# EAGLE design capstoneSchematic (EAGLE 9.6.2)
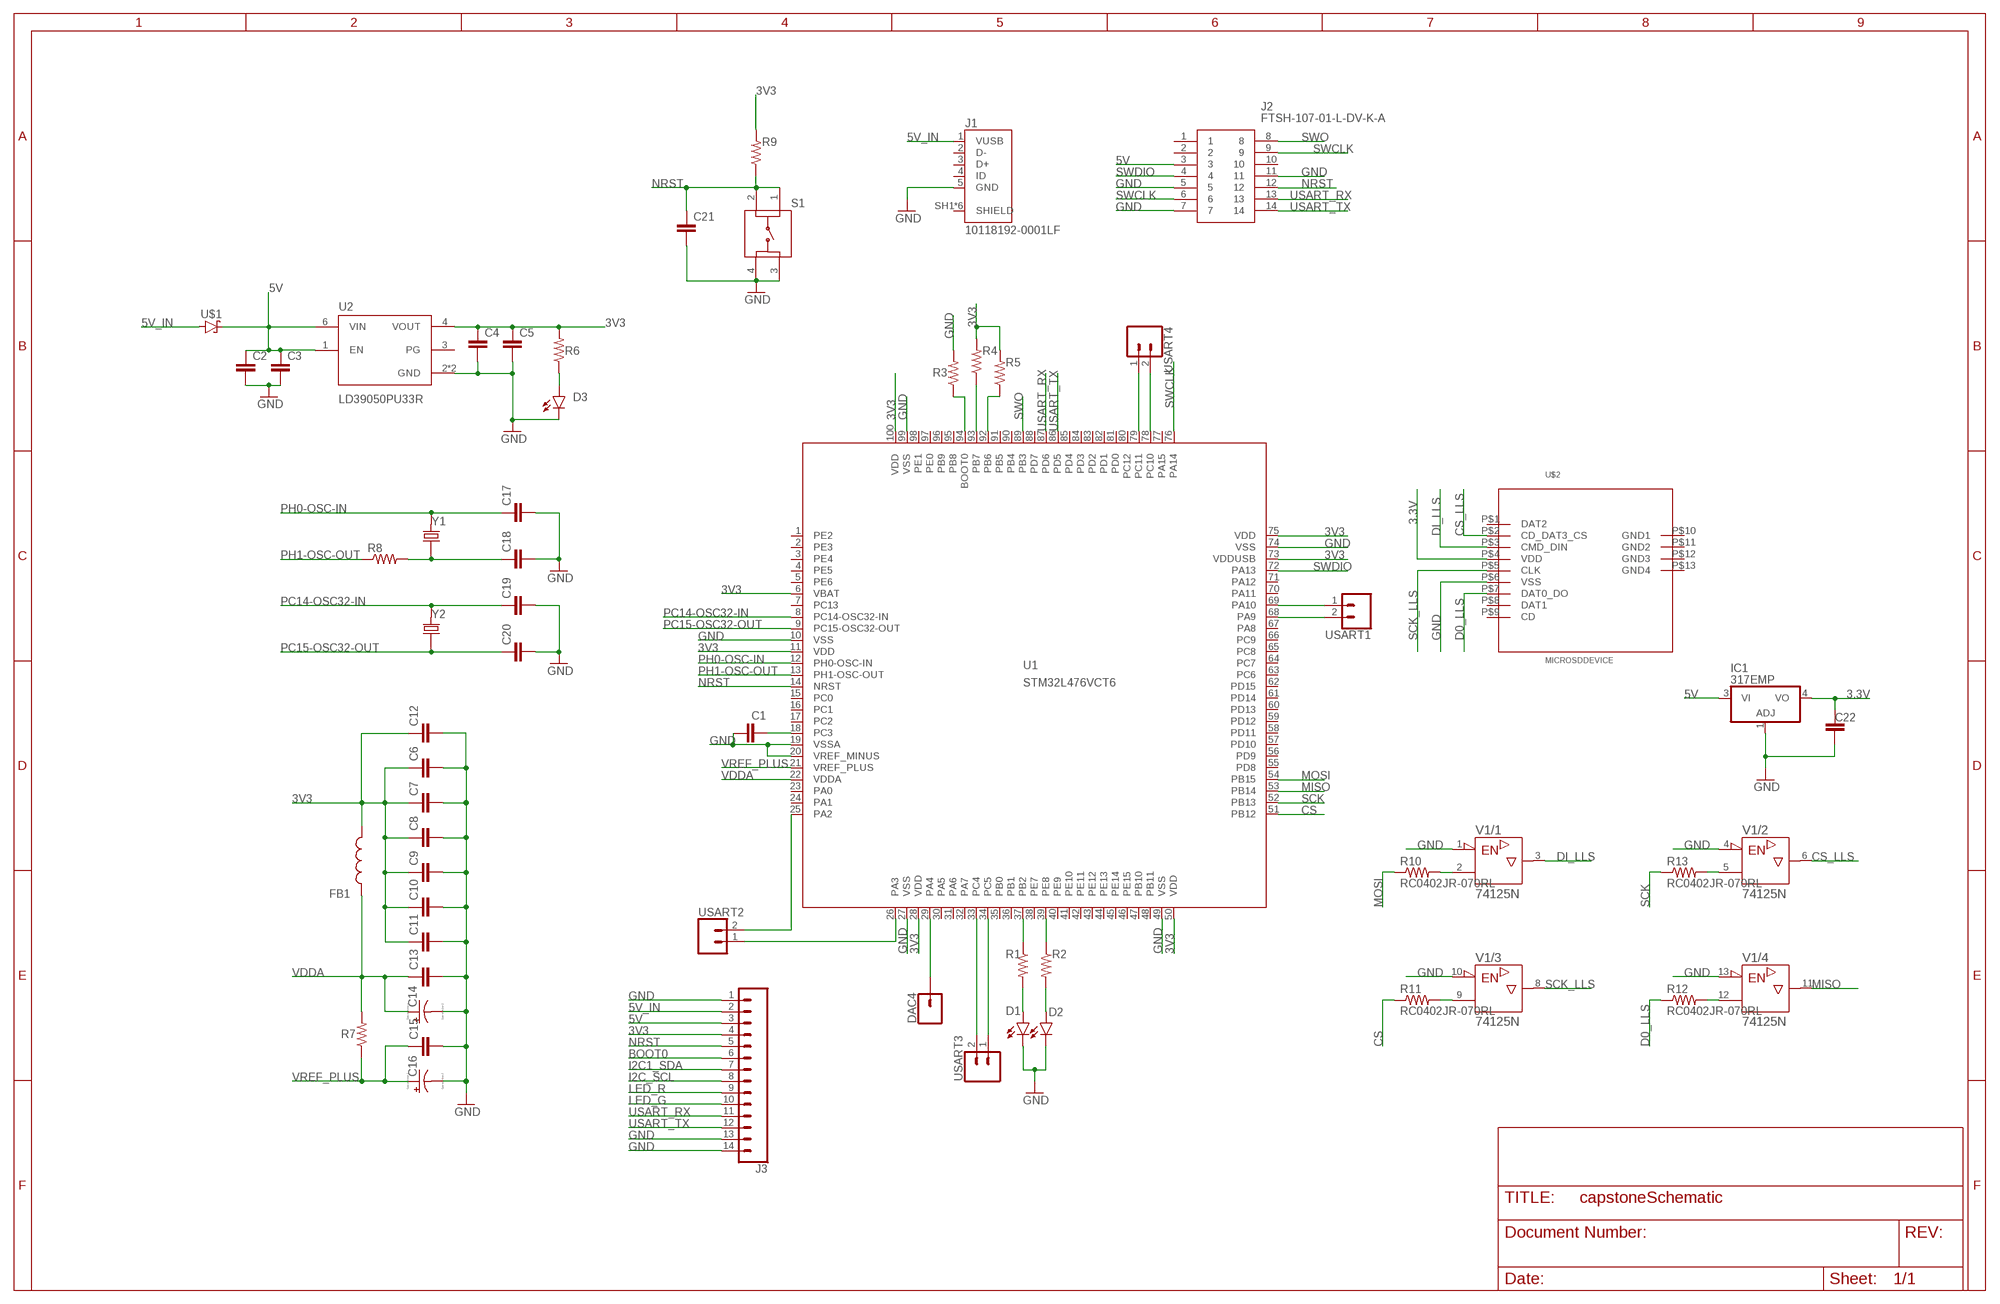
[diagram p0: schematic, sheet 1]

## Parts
C1  CC0603KRX5R7BB105  [CAPC1608X90]
C2  CC0603KRX5R7BB105  [CAPC1608X90]
C3  CC0402KRX7R7BB104  [CAPC1005X55N]
C4  CC0603KRX5R7BB105  [CAPC1608X90]
C5  CC0402KRX7R7BB104  [CAPC1005X55N]
C6  CC0402KRX7R7BB104  [CAPC1005X55N]
C7  CC0402KRX7R7BB104  [CAPC1005X55N]
C8  CC0402KRX7R7BB104  [CAPC1005X55N]
C9  CC0402KRX7R7BB104  [CAPC1005X55N]
C10  CC0402KRX7R7BB104  [CAPC1005X55N]
C11  CC0402KRX7R7BB104  [CAPC1005X55N]
C12  CC0603KRX5R7BB105  [CAPC1608X90]
C13  CC0402KRX7R7BB104  [CAPC1005X55N]
C14  TAJA105K016RNJ  [CAPPM3216X180N]
C15  CC0402KRX7R7BB104  [CAPC1005X55N]
C16  TAJA105K016RNJ  [CAPPM3216X180N]
C17  CC0402JRNPO9BN200  [CAPC1005X55N]
C18  CC0402JRNPO9BN200  [CAPC1005X55N]
C19  CC0402CRNPO9BN4R7  [CAPC1005X55N]
C20  CC0402CRNPO9BN4R7  [CAPC1005X55N]
C21  CC0402KRX7R7BB104  [CAPC1005X55N]
C22  C  (no package)
D1  SML-P12MTT86  [LED_SML-P11UTT86R]
D2  SML-P12MTT86  [LED_SML-P11UTT86R]
D3  SML-P12MTT86  [LED_SML-P11UTT86R]
DAC4  CONN_01  [1X01]
FB1  BK1608HS601-T  [BEADC1608X95N]
IC1  317EMP  [SOT223]
J1  10118192-0001LF  [AMPHENOL_10118192-0001LF]
J2  FTSH-107-01-L-DV-K-A  [FTSH10701LDVKA]
J3  CONN_14  [1X14]
R1  RC0402FR-071KL  [RESC1005X40N]
R2  RC0402FR-071KL  [RESC1005X40N]
R3  RC0402FR-071KL  [RESC1005X40N]
R4  RC0402FR-071KL  [RESC1005X40N]
R5  RC0402FR-071KL  [RESC1005X40N]
R6  RC0402FR-071KL  [RESC1005X40N]
R7  RC0402FR-071KL  [RESC1005X40N]
R8  RC0402FR-072KL  [RESC1005X40N]
R9  RC0402FR-0710KL  [RESC1005X40N]
R10  RC0402JR-070RL  [RESC1005X40]
R11  RC0402JR-070RL  [RESC1005X40]
R12  RC0402JR-070RL  [RESC1005X40]
R13  RC0402JR-070RL  [RESC1005X40]
S1  LL3301FF065QJ  [LL3301FF065QJ]
U1  STM32L476VCT6  [LQFP100_14X14]
U2  LD39050PU33R  [SON95P300X300X100-7N]
U$1  STPS1L30A  [DIOM5226X223N]
U$2  MICROSDDEVICE  [MICROSD]
USART1  CONN_02  [1X02]
USART2  CONN_02  [1X02]
USART3  CONN_02  [1X02]
USART4  CONN_02  [1X02]
V1  74125N  [DIL14]
Y1  ABLS-8.000MHZ-B2-T  [XTAL_ABLS-8.000MHZ-B2-T]
Y2  ECS-.327-12.5-12QS-TR  [XTAL_ECS-.327-12.5-12QS-TR]

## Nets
3.3V: C22.1 IC1.4(VO) U$2.P$4(VDD)
3V3: C4.1 C5.1 C6.1 C7.1 C8.1 C9.1 C10.1 C11.1 C12.1 FB1.2 J3.4 R4.2 R5.2 R6.2 R9.2 U1.6(VBAT) U1.11(VDD) U1.28(VDD) U1.50(VDD) U1.73(VDDUSB) U1.75(VDD) U1.100(VDD) U2.4(VOUT)
5V: C2.1 C3.1 IC1.3(VI) J2.3 J3.3 U2.1(EN) U2.6(VIN) U$1.1(C)
5V_IN: J1.1(VUSB) J3.2 U$1.2(A)
BOOT0: J3.6
CS: R11.1 U1.51(PB12)
CS_LLS: U$2.P$2(CD_DAT3_CS) V1.6(/2:Y)
D0_LLS: R12.1 U$2.P$7(DAT0_DO)
DI_LLS: U$2.P$3(CMD_DIN) V1.3(/1:Y)
GND: C1.1 C2.2 C3.2 C4.2 C5.2 C6.2 C7.2 C8.2 C9.2 C10.2 C11.2 C12.2 C13.2 C14.C(-) C15.2 C16.C(-) C17.2 C18.2 C19.2 C20.2 C21.2 C22.2 D1.C D2.C D3.C IC1.1(ADJ) J1.5(GND) J2.5 J2.7 J2.11 J3.1 J3.13 J3.14 R3.2 S1.3 S1.4 U1.10(VSS) U1.19(VSSA) U1.20(VREF_MINUS) U1.27(VSS) U1.49(VSS) U1.74(VSS) U1.99(VSS) U2.2(GND) U2.7(GND) U$2.P$6(VSS) V1.1(/1:!G) V1.4(/2:!G) V1.10(/3:!G) V1.13(/4:!G)
I2C1_SDA: J3.7
I2C_SCL: J3.8
LED_G: J3.10
LED_R: J3.9
MISO: U1.53(PB14) V1.11(/4:Y)
MOSI: R10.1 U1.54(PB15)
N$1: R2.1 U1.39(PE8)
N$2: R1.1 U1.37(PB2)
N$3: D1.A R1.2
N$4: D2.A R2.2
N$5: R3.1 U1.94(BOOT0)
N$6: R4.1 U1.93(PB7)
N$7: R5.1 U1.92(PB6)
N$8: D3.A R6.1
N$9: U1.33(PC4) USART3.2
N$10: C1.2 U1.18(PC3)
N$11: U1.34(PC5) USART3.1
N$12: C18.1 R8.2 Y1.1
N$13: R10.2 V1.2(/1:A)
N$14: U1.78(PC10) USART4.2
N$15: R11.2 V1.9(/3:A)
N$16: U1.79(PC11) USART4.1
N$17: R13.2 V1.5(/2:A)
N$18: DAC4.1 U1.29(PA4)
N$19: U1.69(PA10) USART1.1
N$20: U1.68(PA9) USART1.2
N$21: R12.2 V1.12(/4:A)
N$22: U1.25(PA2) USART2.2
N$23: U1.26(PA3) USART2.1
NRST: C21.1 J2.12 J3.5 R9.1 S1.1 S1.2 U1.14(NRST)
PC14-OSC32-IN: C19.1 U1.8(PC14-OSC32-IN) Y2.2
PC15-OSC32-OUT: C20.1 U1.9(PC15-OSC32-OUT) Y2.1
PH0-OSC-IN: C17.1 U1.12(PH0-OSC-IN) Y1.2
PH1-OSC-OUT: R8.1 U1.13(PH1-OSC-OUT)
SCK: R13.1 U1.52(PB13)
SCK_LLS: U$2.P$5(CLK) V1.8(/3:Y)
SWCLK: J2.6 J2.9 U1.76(PA14)
SWDIO: J2.4 U1.72(PA13)
SWO: J2.8 U1.89(PB3)
USART_RX: J2.13 J3.11 U1.87(PD6)
USART_TX: J2.14 J3.12 U1.86(PD5)
VDDA: C13.1 C14.A(+) FB1.1 R7.2 U1.22(VDDA)
VREF_PLUS: C15.1 C16.A(+) R7.1 U1.21(VREF_PLUS)
Unconnected: J1.2(D-) J1.3(D+) J1.4(ID) J1.SH1(SHIELD) J1.SH2(SHIELD) J1.SH3(SHIELD) J1.SH4(SHIELD) J1.SH5(SHIELD) J1.SH6(SHIELD) J2.1 J2.2 J2.10 U1.1(PE2) U1.2(PE3) U1.3(PE4) U1.4(PE5) U1.5(PE6) U1.7(PC13) U1.15(PC0) U1.16(PC1) U1.17(PC2) U1.23(PA0) U1.24(PA1) U1.30(PA5) U1.31(PA6) U1.32(PA7) U1.35(PB0) U1.36(PB1) U1.38(PE7) U1.40(PE9) U1.41(PE10) U1.42(PE11) U1.43(PE12) U1.44(PE13) U1.45(PE14) U1.46(PE15) U1.47(PB10) U1.48(PB11) U1.55(PD8) U1.56(PD9) U1.57(PD10) U1.58(PD11) U1.59(PD12) U1.60(PD13) U1.61(PD14) U1.62(PD15) U1.63(PC6) U1.64(PC7) U1.65(PC8) U1.66(PC9) U1.67(PA8) U1.70(PA11) U1.71(PA12) U1.77(PA15) U1.80(PC12) U1.81(PD0) U1.82(PD1) U1.83(PD2) U1.84(PD3) U1.85(PD4) U1.88(PD7) U1.90(PB4) U1.91(PB5) U1.95(PB8) U1.96(PB9) U1.97(PE0) U1.98(PE1) U2.3(PG) U$2.P$1(DAT2) U$2.P$8(DAT1) U$2.P$9(CD) U$2.P$10(GND1) U$2.P$11(GND2) U$2.P$12(GND3) U$2.P$13(GND4)

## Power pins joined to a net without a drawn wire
+UB: V1.14(/+UB:+UB)
-UB: V1.7(/-UB:-UB)

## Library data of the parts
C1 C2 C4 C12 = ce-capstone:CC0603KRX5R7BB105: CAPACITOR CERAMIC, 1µF, 10V, X5R, 0603; Dielectric Characteristic:X5R; Capacitance:1µF; Capacitance Tolerance:± 10%; Voltage Rating:16V; Temperature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; DESCRIPTION: 1µF ±10% 16V Ceramic Capacitor X5R 0603 _1608 Metric_; DIGI-KEY_PART_NUMBER: 311-1444-1-ND; DIGI-KEY_PURCHASE_URL: https://www.digikey.com/product-detail/en/yageo/CC0603KRX5R7BB105/311-1444-1-ND/2833750?utm_source=snapeda&utm_medium=aggregator&utm_campaign=symbol; MF: Yageo; MP: CC0603KRX5R7BB105; PACKAGE: 0603 Yageo
C3 C5-C11 C13 C15 C21 = ce-capstone:CC0402KRX7R7BB104: .1UF 16V 10% 0402; DESCRIPTION: 0.1µF ±10% 16V Ceramic Capacitor X7R 0402 _1005 Metric_; DIGI-KEY_PART_NUMBER: 311-1338-1-ND; DIGI-KEY_PURCHASE_URL: https://www.digikey.com/product-detail/en/yageo/CC0402KRX7R7BB104/311-1338-1-ND/2103122?utm_source=snapeda&utm_medium=aggregator&utm_campaign=symbol; MF: Yageo; MP: CC0402KRX7R7BB104; PACKAGE: 0402 Yageo
C14 C16 = ce-capstone:TAJA105K016RNJ: Capacitor tantalum TAJ 1206 1uF 16V AVX 1uF SMD Solid MnO2 Tantalum Electrolytic Capacitor, 16 V dc +/-10%, TAJ Series; ALLIED_NUMBER: 70474975; ALLIED_PRICE-STOCK: https://www.alliedelec.com/avx-taja105k016r/70474975/; DESCRIPTION: Capacitor tantalum TAJ 1206 1uF 16V AVX 1uF SMD Solid MnO2 Tantalum Electrolytic Capacitor, 16 V dc +/-10%, TAJ Series; HEIGHT: 1.8mm; MANUFACTURER_NAME: AVX; MANUFACTURER_PART_NUMBER: TAJA105K016RNJ; MOUSER_PART_NUMBER: 581-TAJA105K016RNJ; MOUSER_PRICE-STOCK: https://www.mouser.com/Search/Refine.aspx?Keyword=581-TAJA105K016R; RS_PART_NUMBER: 6992804P; RS_PRICE-STOCK: http://uk.rs-online.com/web/p/products/6992804P
C17 C18 = ce-capstone:CC0402JRNPO9BN200: CAPACITOR CERAMIC 20PF 50V, C0G, 0402; Dielectric Characteristic:C0G / NP0; Capacitance:20pF; Capacitance Tolerance:± 5%; Voltage Rating:50V; Capacitor Case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; DESCRIPTION: 20pF ±5% 50V Ceramic Capacitor C0G, NP0 0402 _1005 Metric_; DIGI-KEY_PART_NUMBER: 311-1417-1-ND; DIGI-KEY_PURCHASE_URL: https://www.digikey.com/product-detail/en/yageo/CC0402JRNPO9BN200/311-1417-1-ND/2833723?utm_source=snapeda&utm_medium=aggregator&utm_campaign=symbol; MF: Yageo; MP: CC0402JRNPO9BN200; PACKAGE: 0402 Yageo
C19 C20 = ce-capstone:CC0402CRNPO9BN4R7: 0402 4.7 pF 50 V ±0.25 pF Tolerance NP0 SMT Multilayer Ceramic Capacitor; DESCRIPTION: 4.7pF ±0.25pF 50V Ceramic Capacitor C0G, NP0 0402 _1005 Metric_; DIGI-KEY_PART_NUMBER: 311-1367-1-ND; DIGI-KEY_PURCHASE_URL: https://www.digikey.com/product-detail/en/yageo/CC0402CRNPO9BN4R7/311-1367-1-ND/2103151?utm_source=snapeda&utm_medium=aggregator&utm_campaign=symbol; MF: Yageo; MP: CC0402CRNPO9BN4R7; PACKAGE: 0402 Yageo
C22 = ngspice-simulation:C: CAPACITOR
D1-D3 = ce-capstone:SML-P12MTT86: SML-P1 Series Red 0402 Clear 60 mcd 2 V Surface Mount PICOLED LED; AVAILABILITY: Unavailable; DESCRIPTION: Green 572nm LED Indication - Discrete 2V 0402 _1006 Metric_; MF: Rohm; MP: SML-P12MTT86; PACKAGE: 0402 Rohm; PRICE: None
DAC4 = SparkFun-Connectors:CONN_01: Single connection point. Often used as Generic Header-pin footprint for 0.1 inch spaced/style header connections
FB1 = ce-capstone:BK1608HS601-T: Ferrite Chip Bead(Lead Free); DESCRIPTION: Ferrite Chip Bead(Lead Free); HEIGHT: 0.95mm; MANUFACTURER_NAME: Taiyo Yuden; MANUFACTURER_PART_NUMBER: BK1608HS601-T
IC1 = linear:*317: Positive VOLTAGE REGULATOR
J1 = ce-capstone:10118192-0001LF: Single Port 5 Contact Horizontal Right Angle Shielded Micro B USB 2.0 Connector; AVAILABILITY: Unavailable; DESCRIPTION: USB - micro B USB 2.0 Receptacle Connector 5 Position Surface Mount, Right Angle; MF: Amphenol ICC; MP: 10118192-0001LF; PACKAGE: None; PRICE: None
J2 = ce-capstone:FTSH-107-01-L-DV-K-A: Headers & Wire Housings .050" Micro Terminal Strip Source: Datasheet; DESCRIPTION: Headers & Wire Housings .050" Micro Terminal Strip; HEIGHT: 5.97mm; MANUFACTURER_NAME: SAMTEC; MANUFACTURER_PART_NUMBER: FTSH-107-01-L-DV-K-A; MOUSER_PART_NUMBER: 200-FTSH10701LDVKA; MOUSER_PRICE-STOCK: https://www.mouser.com/Search/Refine.aspx?Keyword=200-FTSH10701LDVKA
J3 = SparkFun-Connectors:CONN_14: Multi connection point. Often used as Generic Header-pin footprint for 0.1 inch spaced/style header connections On any of the 0.1 inch spaced packages, you can populate with these: Break Away Headers - Straight (PRT-00116) Break Away Male Headers - Right Angle (PRT-00553) Female Headers (PRT-00115)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
R1-R7 = ce-capstone:RC0402FR-071KL: RES SMD 1k OHM 1% 1/16W 0402; DESCRIPTION: 510 Ohms ±1% 0.063W, 1/16W Chip Resistor 0402 _1005 Metric_ Moisture Resistant Thick Film; DIGI-KEY_PART_NUMBER: 311-510LRCT-ND; DIGI-KEY_PURCHASE_URL: https://www.digikey.com/product-detail/en/yageo/RC0402FR-07510RL/311-510LRCT-ND/729579?utm_source=snapeda&utm_medium=aggregator&utm_campaign=symbol; MF: Yageo; MP: RC0402FR-07510RL; PACKAGE: 1005 Panasonic Electronic Components
R8 = ce-capstone:RC0402FR-072KL: RES SMD 2k OHM 1% 1/16W 0402; DESCRIPTION: 510 Ohms ±1% 0.063W, 1/16W Chip Resistor 0402 _1005 Metric_ Moisture Resistant Thick Film; DIGI-KEY_PART_NUMBER: 311-510LRCT-ND; DIGI-KEY_PURCHASE_URL: https://www.digikey.com/product-detail/en/yageo/RC0402FR-07510RL/311-510LRCT-ND/729579?utm_source=snapeda&utm_medium=aggregator&utm_campaign=symbol; MF: Yageo; MP: RC0402FR-07510RL; PACKAGE: 1005 Panasonic Electronic Components
R9 = ce-capstone:RC0402FR-0710KL: RES SMD 10k OHM 1% 1/16W 0402; DESCRIPTION: 510 Ohms ±1% 0.063W, 1/16W Chip Resistor 0402 _1005 Metric_ Moisture Resistant Thick Film; DIGI-KEY_PART_NUMBER: 311-510LRCT-ND; DIGI-KEY_PURCHASE_URL: https://www.digikey.com/product-detail/en/yageo/RC0402FR-07510RL/311-510LRCT-ND/729579?utm_source=snapeda&utm_medium=aggregator&utm_campaign=symbol; MF: Yageo; MP: RC0402FR-07510RL; PACKAGE: 1005 Panasonic Electronic Components
R10-R13 = ce-capstone:RC0402JR-070RL: RC Series 0402 62.5 mW 0 Ohms 5% ±200 ppm/°C SMT Thick Film Chip Resistor; AVAILABILITY: Unavailable; DESCRIPTION: 0 Ohms Jumper 0.063W, 1/16W Chip Resistor 0402 _1005 Metric_ Moisture Resistant Thick Film; MF: Yageo; MP: RC0402JR-070RL; PACKAGE: 0402 Yageo; PRICE: None
S1 = ce-capstone:LL3301FF065QJ: Pushbutton Switches 50mA 12VDC F065 7.0mm J-Lead Source: Datasheet; DESCRIPTION: Pushbutton Switches 50mA 12VDC F065 7.0mm J-Lead; HEIGHT: 7.3mm; MANUFACTURER_NAME: E-Switch; MANUFACTURER_PART_NUMBER: LL3301FF065QJ; MOUSER_PART_NUMBER: 612-LL3301FF065QJ; MOUSER_PRICE-STOCK: https://www.mouser.com/Search/Refine.aspx?Keyword=612-LL3301FF065QJ
U1 = ce-capstone:STM32L476V*: STM32L476VX LQFP100 Datasheet STM32L476XX; FARNELL: 2518171; FLASH: 256kB; SRAM: 128kB
U2 = ce-capstone:LD39050PU33R: LD39050 Series 500 mA 3.3 V Fixed Low Noise LDO Voltage Regulator - DFN-6; AVAILABILITY: Unavailable; DESCRIPTION: Linear Voltage Regulator IC 1 Output 500mA 6-DFN _3x3_; MF: STMicroelectronics; MP: LD39050PU33R; PACKAGE: DFN-6 STMicroelectronics; PRICE: None
U$1 = ce-capstone:STPS1L30A
U$2 = MicroSDFootprint:MICROSDDEVICE
USART1-USART4 = SparkFun-Connectors:CONN_02: Multi connection point. Often used as Generic Header-pin footprint for 0.1 inch spaced/style header connections
V1 = 74ttl-din:74*125: Quad bus BUFFER, 3-state
Y1 = ce-capstone:ABLS-8.000MHZ-B2-T: Crystal 8MHz Â±20ppm (Tol) Â±50ppm (Stability) 18pF FUND 80Ohm 2-Pin HC-49/US SMD T/R; AVAILABILITY: Unavailable; DESCRIPTION: 8MHz ±20ppm Crystal 18pF 80 Ohms HC-49/US; MF: Abracon LLC; MP: ABLS-8.000MHZ-B2; PACKAGE: HC-49/US Abracon LLC; PRICE: None
Y2 = ce-capstone:ECS-.327-12.5-12QS-TR: SMD CRYSTAL 32.768 KHz; AVAILABILITY: Unavailable; DESCRIPTION: 32.768kHz ±20ppm Crystal 12.5pF 90 kOhms 2-SMD, No Lead; MF: ECS Inc.; MP: ECS-.327-12.5-12QS-TR; PACKAGE: SMD-2 ECS International; PRICE: None

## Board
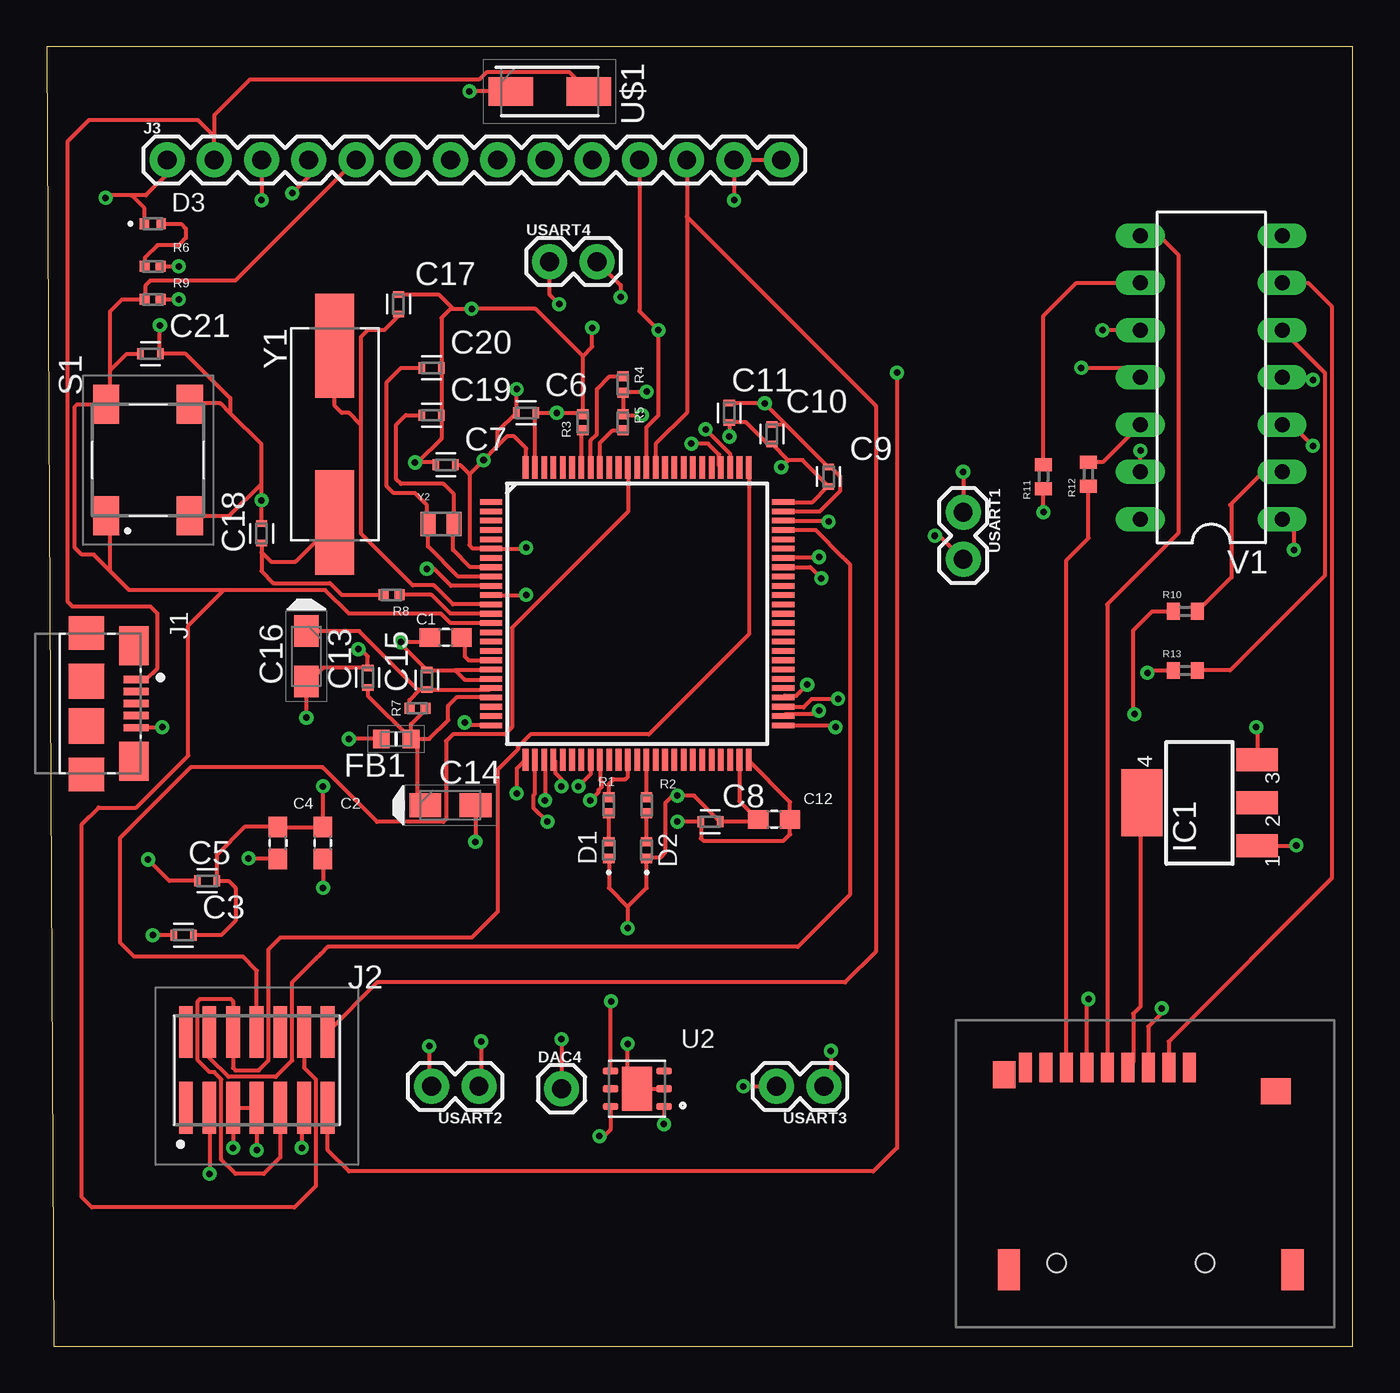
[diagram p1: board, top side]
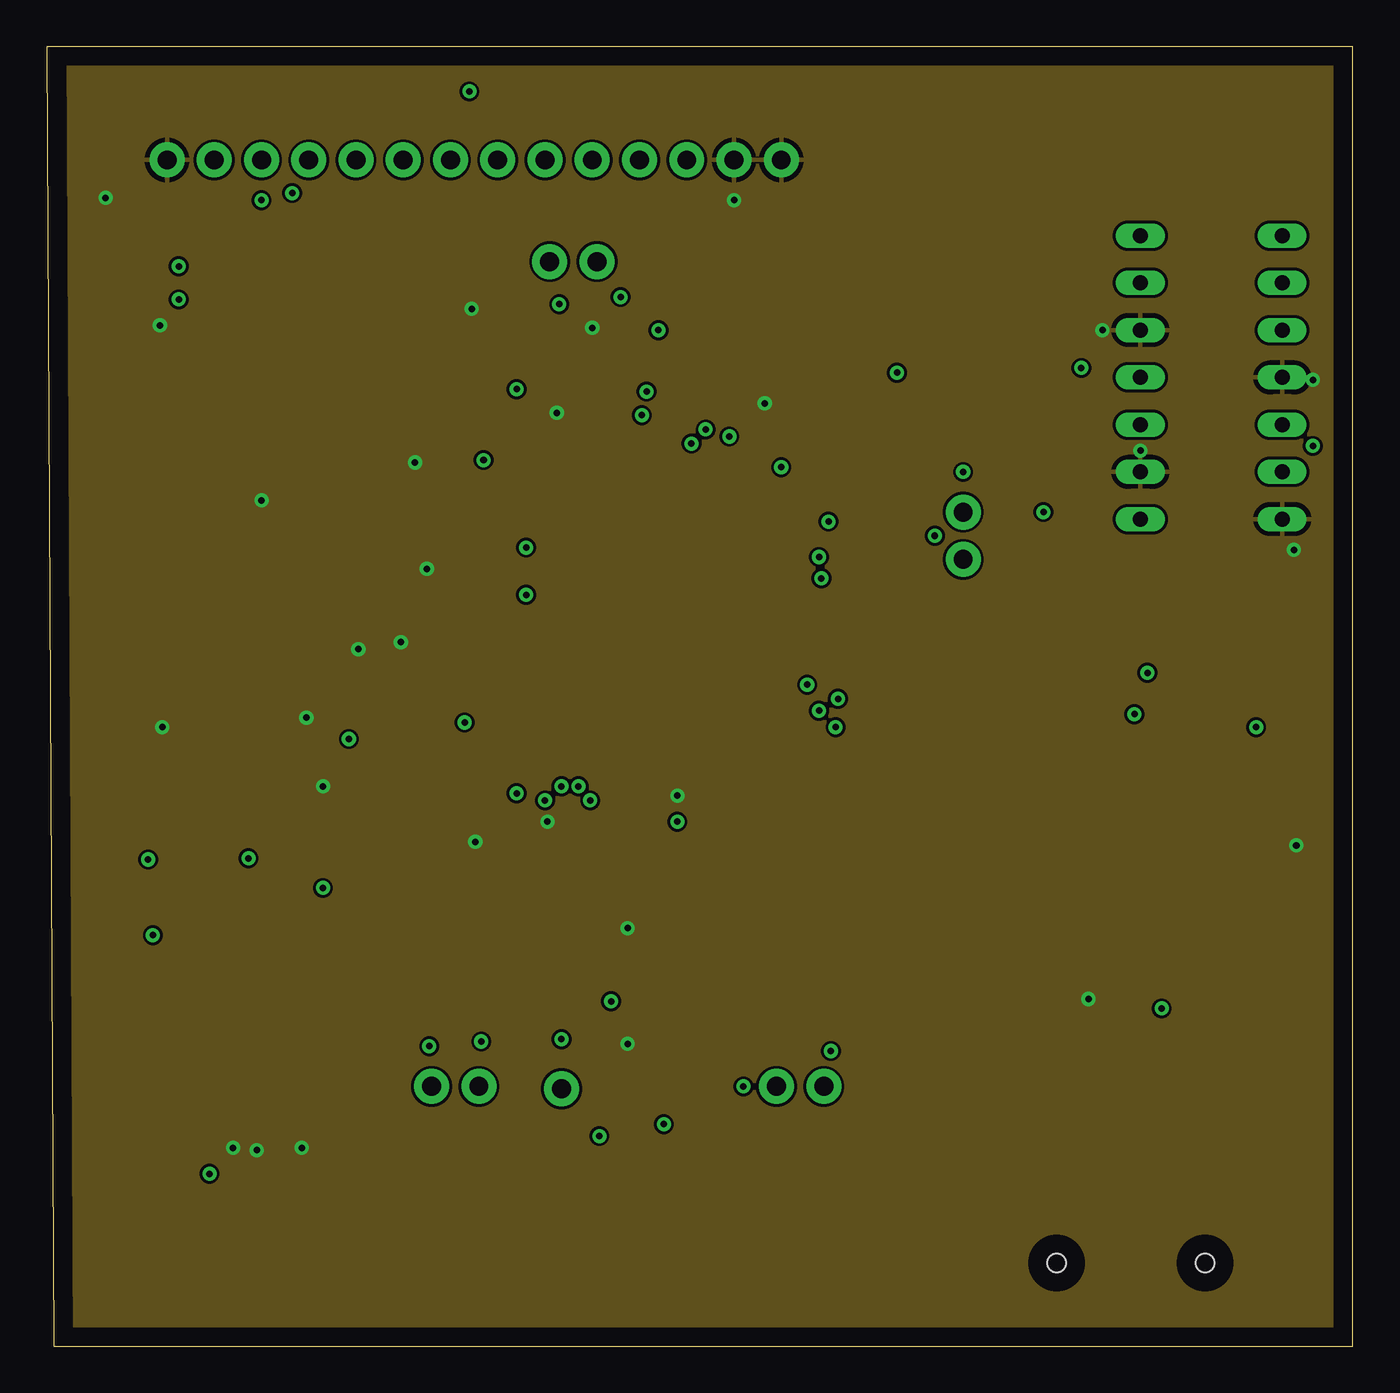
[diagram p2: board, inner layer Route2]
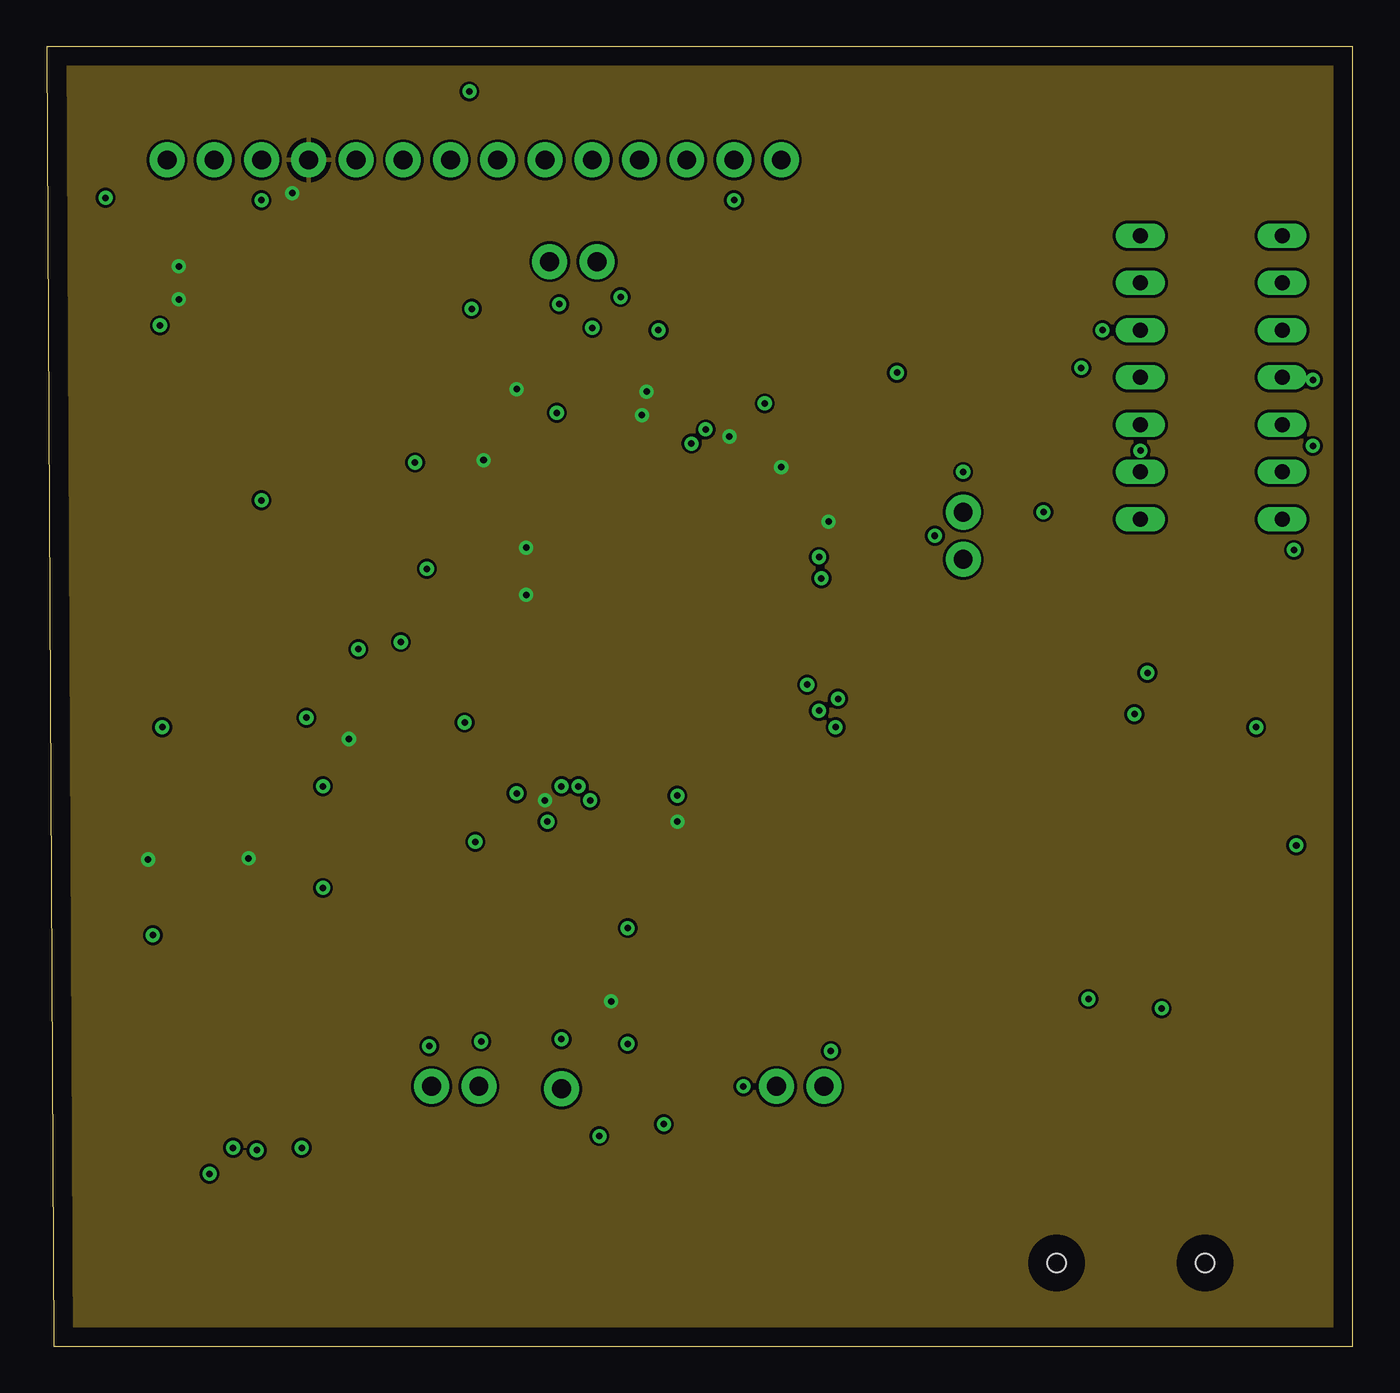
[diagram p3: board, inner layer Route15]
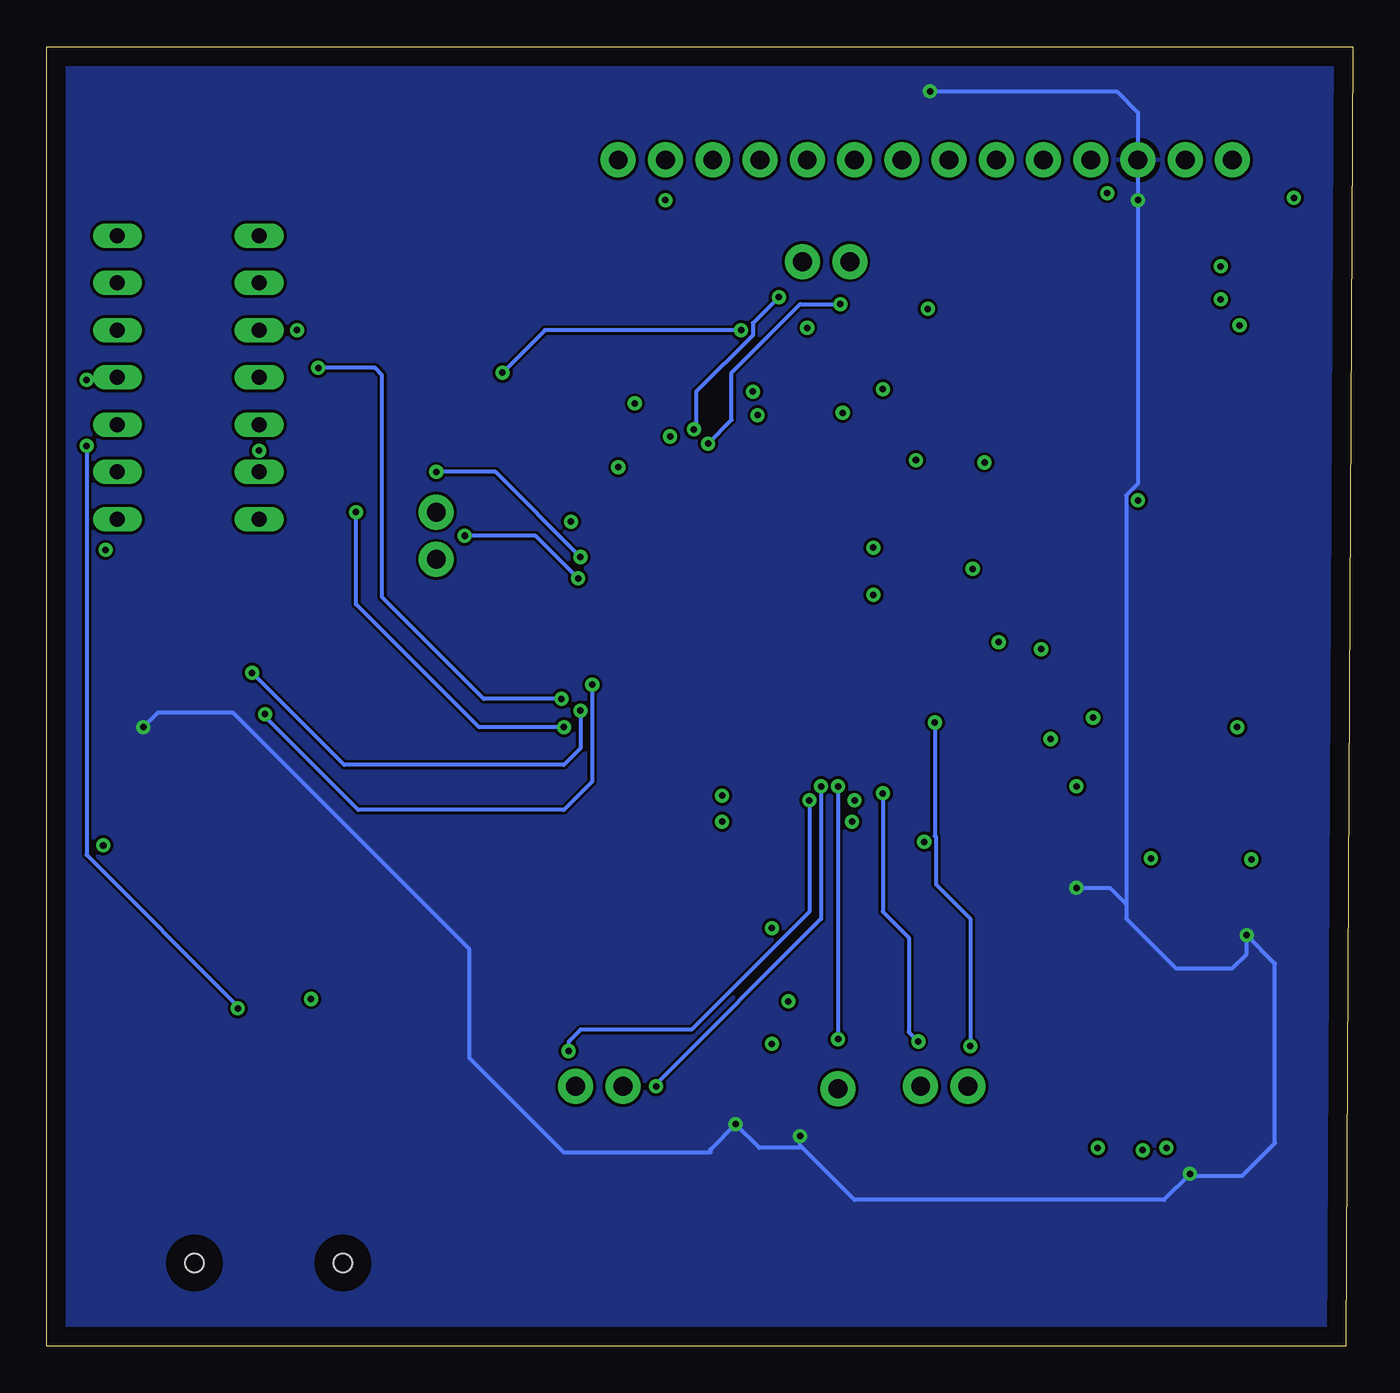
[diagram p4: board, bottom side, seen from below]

Size 70.23 x 69.85 mm. Coordinates in mm from the lower left corner, seen from the top.
Outline: 0.38,0 70.23,0 70.23,69.85 0,69.85 0.38,0
Copper layers (1+2*15+16): Top 0.035mm / dielectric 1.5mm / Route2 0.035mm / dielectric 0.15mm / Route15 0.035mm / dielectric 0.2mm / Bottom 0.035mm
Design rules "default *": minimum track width 8mil, minimum drill 0.35mm, track to track 6mil, track to pad 6mil, pad to pad 6mil, via to via 6mil, smd to smd 6mil, copper to edge 40mil, drill to drill 6mil, minimum pad ring 10mil, minimum via ring 8mil, stop-mask expansion 4mil, vias tented up to drill 0mil, thermal gap 10mil

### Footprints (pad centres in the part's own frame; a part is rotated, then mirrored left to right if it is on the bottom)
CAPC1608X90 = smd 1.1 x 1: 1 -0.85,0; 2 0.85,0
CAPC1005X55N = smd 0.35 x 0.6: 1 -0.525,0; 2 0.525,0
CAPPM3216X180N = smd 1.7 x 1.3: A -1.35,0; C 1.35,0
LED_SML-P11UTT86R = smd 0.5 x 0.6: A 0.45,0; C -0.45,0
1X01 = drill 1.016 pad 1.88: 1 0,0
BEADC1608X95N = smd 0.9 x 1: 1 -0.8,0; 2 0.8,0
SOT223 = smd 1.219 x 2.235: 1 -2.311,-3.099; 2 0,-3.099; 3 2.311,-3.099 | smd 3.6 x 2.2: 4 0,3.099
AMPHENOL_10118192-0001LF = smd 0.4 x 1.35: 1 -1.3,0; 2 -0.65,0; 3 0,0; 4 0.65,0; 5 1.3,0 | smd 2.1 x 1.6: SH1 -3.1,-0.125; SH2 3.1,-0.125 | smd 1.8 x 1.9: SH3 -3.8,-2.675; SH6 3.8,-2.675 | smd 1.9 x 1.9: SH4 -1.2,-2.675; SH5 1.2,-2.675
FTSH10701LDVKA = smd 0.74 x 2.79: 1 -3.81,-2.035; 2 -3.81,2.035; 3 -2.54,-2.035; 4 -2.54,2.035; 5 -1.27,-2.035; 6 -1.27,2.035; 7 0,-2.035; 8 0,2.035; 9 1.27,-2.035; 10 1.27,2.035; 11 2.54,-2.035; 12 2.54,2.035; 13 3.81,-2.035; 14 3.81,2.035
1X14 = drill 1.016 pad 1.88: 1 0,0; 2 2.54,0; 3 5.08,0; 4 7.62,0; 5 10.16,0; 6 12.7,0; 7 15.24,0; 8 17.78,0; 9 20.32,0; 10 22.86,0; 11 25.4,0; 12 27.94,0; 13 30.48,0; 14 33.02,0
RESC1005X40N = smd 0.54 x 0.6: 1 -0.432,0; 2 0.432,0
RESC1005X40 = smd 0.7 x 0.9: 1 -0.65,0; 2 0.65,0
LL3301FF065QJ = smd 2.1 x 1.4: 1 -3,2.25; 2 3,2.25; 3 -3,-2.25; 4 3,-2.25
LQFP100_14X14 = smd 1.2 x 0.3: 1 -7.85,6; 2 -7.85,5.5; 3 -7.85,5; 4 -7.85,4.5; 5 -7.85,4; 6 -7.85,3.5; 7 -7.85,3; 8 -7.85,2.5; 9 -7.85,2; 10 -7.85,1.5; 11 -7.85,1; 12 -7.85,0.5; 13 -7.85,0; 14 -7.85,-0.5; 15 -7.85,-1; 16 -7.85,-1.5; 17 -7.85,-2; 18 -7.85,-2.5; 19 -7.85,-3; 20 -7.85,-3.5; 21 -7.85,-4; 22 -7.85,-4.5; 23 -7.85,-5; 24 -7.85,-5.5; 25 -7.85,-6; 51 7.85,-6; 52 7.85,-5.5; 53 7.85,-5; 54 7.85,-4.5; 55 7.85,-4; 56 7.85,-3.5; 57 7.85,-3; 58 7.85,-2.5; 59 7.85,-2; 60 7.85,-1.5; 61 7.85,-1; 62 7.85,-0.5; 63 7.85,0; 64 7.85,0.5; 65 7.85,1; 66 7.85,1.5; 67 7.85,2; 68 7.85,2.5; 69 7.85,3; 70 7.85,3.5; 71 7.85,4; 72 7.85,4.5; 73 7.85,5; 74 7.85,5.5; 75 7.85,6 | smd 0.3 x 1.2: 26 -6,-7.85; 27 -5.5,-7.85; 28 -5,-7.85; 29 -4.5,-7.85; 30 -4,-7.85; 31 -3.5,-7.85; 32 -3,-7.85; 33 -2.5,-7.85; 34 -2,-7.85; 35 -1.5,-7.85; 36 -1,-7.85; 37 -0.5,-7.85; 38 0,-7.85; 39 0.5,-7.85; 40 1,-7.85; 41 1.5,-7.85; 42 2,-7.85; 43 2.5,-7.85; 44 3,-7.85; 45 3.5,-7.85; 46 4,-7.85; 47 4.5,-7.85; 48 5,-7.85; 49 5.5,-7.85; 50 6,-7.85; 76 6,7.85; 77 5.5,7.85; 78 5,7.85; 79 4.5,7.85; 80 4,7.85; 81 3.5,7.85; 82 3,7.85; 83 2.5,7.85; 84 2,7.85; 85 1.5,7.85; 86 1,7.85; 87 0.5,7.85; 88 0,7.85; 89 -0.5,7.85; 90 -1,7.85; 91 -1.5,7.85; 92 -2,7.85; 93 -2.5,7.85; 94 -3,7.85; 95 -3.5,7.85; 96 -4,7.85; 97 -4.5,7.85; 98 -5,7.85; 99 -5.5,7.85; 100 -6,7.85
SON95P300X300X100-7N = smd 0.84 x 0.4: 1 -1.435,0.95; 2 -1.435,0; 3 -1.435,-0.95; 4 1.435,-0.95; 5 1.435,0; 6 1.435,0.95 | smd 1.625 x 2.365: 7 0,0
DIOM5226X223N = smd 2.4 x 1.55: 1 -2.1,0; 2 2.1,0
MICROSD = smd 1.6 x 0.7: P$1 -3.81,1.1; P$2 -3.81,0; P$3 -3.81,-1.1; P$4 -3.81,-2.2; P$5 -3.81,-3.3; P$6 -3.81,-4.4; P$7 -3.81,-5.5; P$8 -3.81,-6.6; P$9 -3.81,-7.7 | smd 1.45 x 1.2: P$10 -3.41,-8.85 | smd 1.4 x 1.6: P$11 -2.54,5.75 | smd 2.2 x 1.2: P$12 7.06,6.65; P$13 7.06,-8.59 | hole 1: 6.69,1.95; 6.69,-6.03
1X02 = drill 1.016 pad 1.88: 1 0,0; 2 2.54,0
DIL14 = drill 0.813 long: 1 -7.62,-3.81; 2 -5.08,-3.81; 3 -2.54,-3.81; 4 0,-3.81; 5 2.54,-3.81; 6 5.08,-3.81; 7 7.62,-3.81; 8 7.62,3.81; 9 5.08,3.81; 10 2.54,3.81; 11 0,3.81; 12 -2.54,3.81; 13 -5.08,3.81; 14 -7.62,3.81
XTAL_ABLS-8.000MHZ-B2-T = smd 5.6 x 2.1: 1 -4.75,0; 2 4.75,0
XTAL_ECS-.327-12.5-12QS-TR = smd 0.8 x 1.3: 1 -0.7,0; 2 0.7,0

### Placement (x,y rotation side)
C1  21.46,38.1 0 top
C2  14.86,27.05 90 top
C3  7.37,22.1 0 top
C4  12.45,27.05 90 top
C5  8.64,25.02 0 top
C6  25.78,50.16 0 top
C7  21.46,47.37 180 top
C8  35.69,28.19 0 top
C9  42.04,46.74 90 top
C10  38.99,49.02 90 top
C11  36.7,50.16 90 top
C12  39.12,28.32 180 top
C13  17.27,35.94 90 top
C14  21.72,29.08 0 top
C15  20.45,35.81 90 top
C16  13.97,37.08 270 top
C17  18.92,56.01 90 top
C18  11.56,43.69 90 top
C19  20.7,50.04 0 top
C20  20.7,52.58 0 top
C21  5.59,53.34 0 top
D1  30.23,26.67 90 top
D2  32.26,26.67 90 top
D3  5.71,60.33 0 top
DAC4  27.69,13.84 0 top
FB1  18.8,32.64 180 top
IC1  61.98,29.21 90 top
J1  4.83,34.54 270 top
J2  11.3,14.86 0 top
J3  6.48,63.75 0 top
R1  30.23,29.08 270 top
R2  32.26,29.08 270 top
R3  28.83,49.66 90 top
R4  30.99,51.69 270 top
R5  30.99,49.66 90 top
R6  5.71,58.04 0 top
R7  19.94,34.29 0 top
R8  18.54,40.39 180 top
R9  5.71,56.26 0 top
R10  61.21,39.5 0 top
R11  53.59,46.74 90 top
R12  56.01,46.86 90 top
R13  61.21,36.32 0 top
S1  5.46,47.62 90 top
U1  31.75,39.37 0 top
U2  31.75,13.84 180 top
U$1  27.05,67.44 0 top
U$2  60.33,11.18 270 top
USART1  49.28,44.83 270 top
USART2  23.24,13.97 180 top
USART3  41.78,13.97 180 top
USART4  27.05,58.29 0 top
V1  62.61,52.07 90 top
Y1  15.49,49.02 90 top
Y2  21.21,44.2 0 top

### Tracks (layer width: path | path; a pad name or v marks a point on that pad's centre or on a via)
3.3V
  Top 0.203: IC1.4 58.8,29.13 58.8,18.26 58.42,17.88 58.42,15.28 U$2.P$4
3V3  (via drill 0.35)
  Top 0.203: 22.73,46.86 22.73,43.05 22.92,42.87 U1.6 25.73,42.87 v25.78,42.93 | 22.73,46.86 v23.5,47.62 24.26,48.39 | 24.26,48.39 24.26,49.17 C6.1 25.26,51.42 v25.27,51.44 | U1.50 37.75,31.46 39.97,29.25 C12.1 39.97,27.52 39.62,27.18 35.31,27.18 35.18,27.3 35.18,28.18 C8.1 v33.91,28.19 | U1.75 41.18,45.37 42.02,46.21 C9.1 40.64,47.61 40.64,47.62 39.88,47.62 | 39.88,47.62 39.86,47.62 C10.1 38.75,48.5 37.59,49.66 36.72,49.66 C11.1 v36.7,48.9 | 39.88,47.62 v39.5,47.24 | FB1.2 v16.26,32.64 | v32.26,51.31 31.04,51.31 R4.2 R5.2 31.04,50.04 v32,50.04 | C7.1 22.23,47.37 22.73,46.86 | U1.100 25.78,47.25 25.78,48.26 25.15,48.9 24.77,48.9 24.26,48.39 | U1.28 26.8,31.47 v26.8,29.34 | U2.4 30.32,18.5 v30.35,18.54 | C5.1 6.6,25.02 v5.46,26.16 | J3.4 14.1,62.87 v13.21,61.98 | R9.2 v7.11,56.26 | R6.2 v7.11,58.04 | U1.73 41.99,44.37 v42.04,44.32 | U1.11 25.77,40.37 v25.78,40.39 | C4.1 10.88,26.2 v10.86,26.23
  pour Route15: 0.76,69.34 69.85,69.34 69.85,0.25 0.76,0.25
5V  (via drill 0.35)
  Top 0.203: U2.1 v33.19,11.94 | U2.6 30.32,11.65 29.97,11.3 v29.72,11.3 | J2.3 v8.76,9.27 | J3.3 v11.56,61.59 | C2.1 v14.86,24.64 | C3.1 v5.71,22.1 | U$1.1 v22.73,67.44 | v65.02,33.27 65.08,33.22 IC1.3
  Bottom 0.203: 12.19,23.75 12.19,45.73 11.56,46.36 v11.56,61.59 11.56,66.29 12.7,67.44 v22.73,67.44 | 12.19,23.75 12.19,22.98 9.53,20.32 6.48,20.32 5.71,21.08 v5.71,22.1 4.19,20.57 4.19,10.92 5.97,9.14 8.89,9.14 | v8.76,9.27 8.89,9.14 | 8.89,9.14 10.16,7.87 26.8,7.87 29.59,10.67 | v29.72,11.3 29.72,10.79 29.59,10.67 | v14.86,24.64 13.08,24.64 12.19,23.75 | 29.59,10.67 31.91,10.67 v33.19,11.94 34.54,10.58 34.54,10.41 42.42,10.41 47.5,15.49 47.5,21.34 60.2,34.04 64.26,34.04 v65.02,33.27
  pour Bottom: 1.14,69.34 69.85,69.34 69.85,0.38 0.89,0.38 0.89,69.47 1.14,69.47
5V_IN
  Top 0.203: J3.2 9.02,65.02 | J1.1 5.3,35.84 5.33,35.81 5.97,36.45 5.97,39.37 5.59,39.75 1.4,39.75 1.14,40.01 1.14,64.77 2.29,65.91 8.13,65.91 9.02,65.02 | U$1.2 28.12,68.47 23.65,68.47 23.25,68.07 10.92,68.07 9.02,66.17 9.02,65.02
CS  (via drill 0.35)
  Top 0.203: U1.51 42.32,33.37 v42.42,33.27 | v53.59,44.83 R11.1
  Bottom 0.203: v42.42,33.27 46.99,33.27 53.59,39.88 v53.59,44.83
CS_LLS
  Top 0.203: V1.6 67.82,57.15 69.09,55.88 69.09,25.15 60.33,16.38 U$2.P$2
D0_LLS
  Top 0.203: U$2.P$7 54.83,42.25 56.01,43.43 R12.1
DI_LLS  (via drill 0.35)
  Top 0.203: V1.3 66.93,49.53 v68.07,48.39 | v59.94,18.16 59.94,17.91 59.23,17.19 U$2.P$3
  Bottom 0.203: v68.07,48.39 68.07,26.42 59.94,18.29 v59.94,18.16
GND  (via drill 0.35)
  Top 0.203: J1.5 4.86,33.27 v6.22,33.27 | v10.03,10.67 J2.5 J2.7 v11.3,10.54 | U1.20 23.86,35.83 22.48,35.83 21.97,36.34 | U1.19 23.87,36.34 21.97,36.34 | 21.97,36.34 C15.2 19.05,37.74 v19.05,37.85 20.36,37.85 C1.1 | U1.99 26.25,50.11 C6.2 v27.43,50.16 28.75,50.16 R3.2 28.83,53.21 | C12.2 38.14,28.19 37.85,28.19 | 37.85,28.19 C8.2 34.81,29.59 v33.91,29.59 33.66,29.59 33.27,29.21 33.27,26.54 33.02,26.29 32.33,26.29 D2.C 32.26,24.64 31.24,23.62 | U1.74 41.57,44.87 42.67,45.97 42.67,46.74 42.15,47.26 C9.2 42.02,47.26 39.73,49.55 | C10.2 39.73,49.55 | 39.73,49.55 v38.61,50.67 36.72,50.67 C11.2 | C14.C 23.07,27.23 23.11,27.18 v23.05,27.12 | C16.C 13.97,35.56 | 13.97,35.56 v13.97,33.78 | D1.C 30.23,24.64 31.24,23.62 | 31.24,23.62 v31.24,22.48 | C18.2 v11.56,45.47 11.56,46.36 | C17.2 21.07,56.53 21.84,55.75 | 21.84,55.75 v22.86,55.75 26.29,55.75 28.83,53.21 | 21.84,55.75 21.72,55.75 21.23,55.26 C20.2 C19.2 21.23,48.79 19.94,47.5 v19.81,47.5 20.81,47.5 C7.2 | S1.3 9.83,44.62 11.56,46.36 | 11.56,46.36 11.56,48.47 9.88,50.14 | U2.2 U2.7 31.24,14.35 v31.24,16.26 | 28.83,53.21 29.34,53.72 v29.34,54.74 | U1.10 21.74,40.87 20.83,41.78 v20.45,41.78 | U1.49 37.25,29.3 37.85,28.7 37.85,28.19 | J2.11 13.84,11.68 13.72,11.56 v13.72,10.67 | C3.2 9.4,22.1 10.16,22.86 10.16,24.64 9.78,25.02 C5.2 9.16,26.42 10.69,27.94 12.41,27.94 C4.2 C2.2 v14.86,30.1 | J3.1 6.48,62.99 5.33,61.85 4.57,61.85 | 4.57,61.85 3.3,61.85 v3.17,61.72 | v6.1,54.86 6.1,53.36 C21.2 7.49,53.34 9.88,50.95 9.88,50.14 | D3.C 5.26,61.16 4.57,61.85 | J3.14 J3.13 v36.96,61.59 | v26.92,28.19 26.16,28.95 26.16,29.6 26.25,29.68 U1.27 | S1.4 7.71,50.67 9.35,50.67 9.88,50.14
  Top 0.203: 13.97,35.56 14.88,36.47 C13.2 17.27,37.08 16.89,37.46 v16.76,37.46 | IC1.1 67.16,26.9 v67.18,26.92 | U$2.P$6 55.92,18.59 v56.01,18.67 | V1.1 67.06,43.82 v67.06,42.8 | V1.10 v56.77,54.61 | V1.13 v58.8,48.13 | V1.4 67.94,52.07 v68.07,51.94
  Route2 0.203: 56.64,54.48 v56.77,54.61
  pour Route2: 0.76,69.34 69.85,69.34 69.85,0.38 0.76,0.38
MISO  (via drill 0.35)
  Top 0.203: U1.53 39.63,34.34 40.69,34.34 41.15,34.8 v42.55,34.8 | v55.63,52.58 58.29,52.58 V1.11
  Bottom 0.203: v42.55,34.8 46.74,34.8 52.2,40.26 52.2,52.2 52.58,52.58 v55.63,52.58
MOSI  (via drill 0.35)
  Top 0.203: U1.54 39.7,34.97 40.3,34.97 40.45,35.12 v40.89,35.56 | v58.48,33.97 58.42,34.04 58.42,38.48 59.44,39.5 R10.1
  Bottom 0.203: v40.89,35.56 40.89,30.35 42.42,28.83 53.47,28.83 58.55,33.91 v58.48,33.97
N$1
  Top 0.203: R2.1 32.25,29.52 U1.39
N$2
  Top 0.203: R1.1 30.23,30.23 30.48,30.48 31.11,30.48 31.25,30.62 U1.37
N$3
  Top 0.203: D1.A R1.2
N$4
  Top 0.203: D2.A R2.2
N$5
  Top 0.203: U1.94 28.75,49.15 R3.1
N$6
  Top 0.203: U1.93 29.25,48.68 29.59,49.02 29.59,51.44 30.28,52.12 R4.1
N$7
  Top 0.203: U1.92 29.75,48.55 30.43,49.23 R5.1
N$8
  Top 0.203: D3.A 7.24,60.33 7.49,60.07 7.49,59.56 7.11,59.18 5.97,59.18 5.28,58.5 R6.1
N$9  (via drill 0.35)
  Top 0.203: U1.33 29.25,30.75 v28.59,30.1 | v37.47,13.97 USART3.2
  Bottom 0.203: v28.59,30.1 28.59,22.97 37.47,14.1 v37.47,13.97
N$10
  Top 0.203: C1.2 22.48,37.93 22.48,37.08 22.69,36.87 U1.18
N$11  (via drill 0.35)
  Top 0.203: U1.34 29.75,30.45 29.84,30.35 29.84,30.06 29.67,29.89 29.67,29.78 v29.23,29.34 | v42.16,15.88 42.16,14.35 USART3.1
  Bottom 0.203: v29.23,29.34 29.23,23.35 35.56,17.02 41.53,17.02 42.16,16.38 v42.16,15.88
N$12
  Top 0.203: C18.1 11.56,42.67 | 11.56,42.67 11.56,41.66 12.19,41.02 15.24,41.02 15.88,40.39 R8.2 | 11.56,42.67 12.06,42.16 13.39,42.16 Y1.1
N$13
  Top 0.203: V1.2 65.41,46.99 63.69,45.27 | 63.69,45.27 63.63,45.21 | 63.69,45.27 63.69,41.32 R10.2
N$14  (via drill 0.35)
  Top 0.203: USART4.2 30.86,57.02 v30.86,56.39 | v35.43,49.28 36.07,48.64 36.07,48.63 36.75,47.95 U1.78
  Bottom 0.203: v30.86,56.39 32.26,54.99 32.26,54.35 35.31,51.3 35.31,49.4 v35.43,49.28
N$15
  Top 0.203: R11.2 53.59,55.37 55.37,57.15 V1.9
N$16  (via drill 0.35)
  Top 0.203: U1.79 36.15,47.32 36.15,47.93 35.56,48.51 v34.67,48.51 | v27.56,56.01 27.05,56.52 USART4.1
  Bottom 0.203: v34.67,48.51 33.4,49.78 33.4,52.32 29.72,56.01 v27.56,56.01
N$17
  Top 0.203: V1.5 68.71,52.32 68.71,41.4 63.63,36.32 R13.2
N$18  (via drill 0.35)
  Top 0.203: U1.29 27.35,31.42 27.35,30.81 27.69,30.48 v27.69,30.1 | v27.69,16.51 DAC4.1
  Bottom 0.203: v27.69,30.1 v27.69,16.51
N$19  (via drill 0.35)
  Top 0.203: U1.69 39.65,42.42 v41.53,42.42 | v49.28,46.99 USART1.1
  Bottom 0.203: v41.53,42.42 46.1,46.99 v49.28,46.99
N$20  (via drill 0.35)
  Top 0.203: U1.68 41.06,41.87 v41.66,41.27 | v47.75,43.56 48.01,43.56 USART1.2
  Bottom 0.203: v41.66,41.27 43.94,43.56 v47.75,43.56
N$21
  Top 0.203: V1.12 56.78,47.51 R12.2
N$22  (via drill 0.35)
  Top 0.203: U1.25 22.63,33.37 v22.48,33.52 | v20.57,16.13 20.57,14.1 USART2.2
  Bottom 0.203: v22.48,33.52 22.48,27.44 22.42,27.38 22.42,24.83 20.57,22.99 v20.57,16.13
N$23  (via drill 0.35)
  Top 0.203: U1.26 25.27,31.04 v25.27,29.72 | v23.37,16.38 23.37,14.1 USART2.1
  Bottom 0.203: v25.27,29.72 25.27,23.37 23.88,21.97 23.88,16.89 v23.37,16.38
NRST
  Top 0.203: U1.14 21.71,38.87 21.21,39.37 16.26,39.37 14.99,40.64 9.53,40.64 | S1.1 3.43,44.84 3.43,41.66 | 9.53,40.64 4.45,40.64 3.43,41.66 | 3.43,41.66 2.54,42.55 1.91,42.55 1.52,42.93 1.52,50.5 1.65,50.62 S1.2 3.43,50.84 3.43,52.45 | 3.43,52.45 4.32,53.34 C21.1 | 3.43,52.45 3.43,55.63 4.06,56.26 R9.1 5.33,56.31 5.33,57.02 5.59,57.28 10.16,57.28 J3.5 | J2.12 13.84,14.99 14.48,14.35 14.48,8.61 13.34,7.47 2.44,7.47 1.91,8 1.91,28.07 2.79,28.96 4.83,28.96 7.62,31.75 7.62,38.73 9.53,40.64
PC14-OSC32-IN
  Top 0.203: U1.8 22.77,41.87 21.84,42.8 21.84,44.13 Y2.2 21.91,45.78 21.34,46.36 19.05,46.36 18.8,46.61 18.8,49.53 19.3,50.04 C19.1
PC15-OSC32-OUT
  Top 0.203: U1.9 22.13,41.37 20.51,42.99 Y2.1 20.51,44.64 20.45,44.7 20.45,45.21 19.81,45.85 18.67,45.85 18.29,46.23 18.29,51.82 19.05,52.58 C20.1
PH0-OSC-IN
  Top 0.203: U1.12 21.85,39.87 20.83,40.89 19.68,40.89 16.89,43.69 16.89,49.53 | C17.1 18.92,55.37 18.16,54.61 17.27,54.61 16.89,54.23 16.89,49.53 | 16.89,49.53 16.26,50.16 15.88,50.16 15.49,50.55 Y1.2
PH1-OSC-OUT
  Top 0.203: U1.13 21.72,39.37 20.7,40.39 R8.1
SCK  (via drill 0.35)
  Top 0.203: U1.52 39.7,33.97 41.33,33.97 v41.53,34.16 | v59.18,36.2 59.31,36.32 R13.1
  Bottom 0.203: v41.53,34.16 41.53,32.13 42.42,31.24 54.23,31.24 v59.18,36.2
SCK_LLS
  Top 0.203: V1.8 59.82,59.69 60.83,58.67 60.83,43.69 57.02,39.88 U$2.P$5
SWCLK
  Top 0.203: J2.9 12.57,10.16 11.68,9.27 10.16,9.27 9.4,10.03 9.4,14.35 9.02,14.73 8.76,14.73 8.13,15.37 8.13,18.54 8.26,18.67 9.91,18.67 10.03,18.54 J2.6 10.03,14.96 10.16,14.83 11.4,14.83 11.94,15.37 11.94,21.34 12.57,21.97 22.86,21.97 24.26,23.37 24.26,30.99 25.35,32.08 25.35,32.23 26.01,32.89 32.38,32.89 37.75,38.26 U1.76
SWDIO
  Top 0.203: U1.72 41.35,43.87 42.8,42.42 42.93,42.29 43.18,42.04 43.18,24.26 40.39,21.46 15.11,21.46 14.73,21.08 14.48,20.83 13.21,19.56 13.21,15.37 12.32,14.48 9.78,14.48 8.76,15.49 J2.4
SWO
  Top 0.203: U1.89 31.25,44.84 25.02,38.61 25.02,33.27 24.64,32.89 21.84,32.89 21.47,32.52 21.47,28.33 21.32,28.18 17.77,28.18 14.86,31.09 14.86,31.12 7.75,31.12 3.94,27.3 3.94,21.72 4.7,20.95 10.54,20.95 11.3,20.19 J2.8
USART_RX  (via drill 0.35)
  Top 0.203: U1.87 32.25,49.39 32.89,50.03 v32.89,54.61 31.88,55.63 J3.11 | v45.72,52.32 45.72,10.67 44.45,9.4 16.26,9.4 15.11,10.54 J2.13
  Bottom 0.203: v32.89,54.61 43.43,54.61 v45.72,52.32
USART_TX
  Top 0.203: U1.86 32.75,48.5 34.42,50.16 34.42,60.71 | J3.12 34.42,60.71 | 34.42,60.71 44.58,50.55 44.58,21.21 42.93,19.56 17.78,19.56 J2.14
VDDA
  Top 0.203: FB1.1 19.94,32.64 | 19.94,32.64 20.57,32.64 21.59,33.66 21.59,34.42 22.04,34.87 U1.22 | FB1.1 17.27,34.96 C13.1 | FB1.1 19.6,33.44 20.37,34.21 R7.2 | C14.A 19.94,29.51 19.94,32.64
VREF_PLUS
  Top 0.203: U1.21 23.82,35.29 C15.1 20.07,35.29 | 20.07,35.29 19.96,35.29 16.81,38.43 C16.A | R7.1 19.51,34.73 20.07,35.29

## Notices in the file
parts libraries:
SparkFun-Connectors: Licensing: Creative Commons ShareAlike 4.0 International - https://creativecommons.org/licenses/by-sa/4.0
